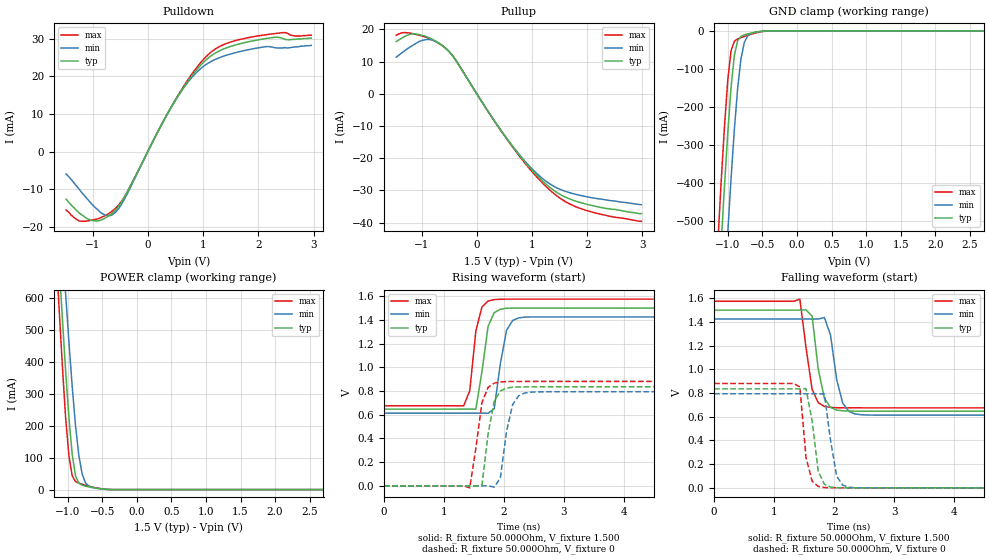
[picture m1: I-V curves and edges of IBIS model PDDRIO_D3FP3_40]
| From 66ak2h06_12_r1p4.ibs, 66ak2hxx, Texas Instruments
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|   Model PDDRIO_D3FP3_40
[Model] PDDRIO_D3FP3_40
Model_type   I/O
Polarity   Non-Inverting
Enable   Active-High
C_comp   3.236pF   3.174pF   3.318pF
C_comp_pullup   516.723fF   493.565fF   544.031fF
C_comp_pulldown 2.715pF   2.675pF   2.769pF
Vinh = 925.000mV
Vinl = 575.000mV
Vmeas = 750.000mV
Vref = 750.000mV
Rref = 50Ohms
Cref = 0pF
[Model Spec]
Vinh   925.000mV   888.000mV   963.000mV
Vinl   575.000mV   538.000mV   613.000mV
Vmeas   750.000mV   713.000mV   788.000mV
Vref   750.000mV   713.000mV   788.000mV
[Temperature Range]   25.000   125.000   -40.000
[Voltage Range]   1.500V   1.425V   1.575V
[GND Clamp Reference]   0.00V   0.00V   0.00V
|[C Comp Corner]
| variable   typ   min   max
|C_comp 3.236pF   3.318pF   3.174pF
|C_comp_pullup 516.723fF   544.031fF   493.565fF
|C_comp_pulldown 2.715pF   2.769pF   2.675pF
[Pulldown Reference]   0.00V   0.00V   0.00V
[POWER Clamp Reference]   1.500V   1.425V   1.575V
[Pullup Reference]   1.500V   1.425V   1.575V
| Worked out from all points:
|   slope of the pulldown table from 0 to 0.225 V, typ, clamps not added: 34.8 ohm
|   slope of the pullup table from 0 to 0.225 V, typ, clamps not added: 37.6 ohm
|   GND clamp passes 1 mA (typ) near -0.49 V on its own axis
|   POWER clamp passes 1 mA (typ) near -0.46 V on its own axis
|   rising waveform, R_fixture 50.000Ohm, V_fixture 1.500: 20-80 % time 145ps typ, 153ps min, 136ps max; typ from 0.647 V to 1.5 V
|   rising waveform, R_fixture 50.000Ohm, V_fixture 0: 20-80 % time 150ps typ, 158ps min, 147ps max; typ from 0 V to 0.836 V
|   falling waveform, R_fixture 50.000Ohm, V_fixture 1.500: 20-80 % time 151ps typ, 165ps min, 148ps max; typ from 1.5 V to 0.647 V
|   falling waveform, R_fixture 50.000Ohm, V_fixture 0: 20-80 % time 134ps typ, 143ps min, 118ps max; typ from 0.836 V to 0 V
[GND Clamp]
-1.48V    -1.918A    -2.181A    -1.764A
-1.145V   -723.4mA   -1.002A    -556.7mA
-1.098V   -563.3mA   -840.4mA   -399.2mA
-1.05V    -410.5mA   -683.3mA   -253.2mA
-1.002V   -269.5mA   -532mA     -130mA
-954.6mV  -149.1mA   -389.4mA   -52.57mA
-906.8mV  -64.77mA   -260.1mA   -27.53mA
-859.1mV  -26.06mA   -151.5mA   -21.41mA
-811.4mV  -14.61mA   -73.73mA   -17.98mA
-715.9mV  -8.245mA   -13.8mA    -12.04mA
-525mV    -1.646mA   -1.444mA   -2.745mA
2.959V    5.126nA    157.9nA    5.129nA
[Power Clamp]
-1.459V   2.052A     2.172A     2.008A
-1.173V   897.3mA    1.113A     766.5mA
-1.125V   714.9mA    943mA      572.9mA
-1.077V   539.1mA    776.9mA    390mA
-1.03V    373.7mA    616.2mA    227.4mA
-981.8mV  225.9mA    463.5mA    105.8mA
-934.1mV  109.7mA    322.9mA    43.29mA
-886.4mV  43.23mA    201.1mA    25.08mA
-838.6mV  20.27mA    107.7mA    20.03mA
-790.9mV  13.81mA    49.43mA    16.8mA
-647.7mV  6.613mA    6.926mA    8.545mA
2.98V     -9.151nA   -320.3nA   -14.09nA
[Pulldown]
-1.48V    -12.7mA    -6mA       -15.6mA
-1.241V   -16.4mA    -10.1mA    -18.5mA
-1.05V    -18.2mA    -13.4mA    -18.4mA
-811.4mV  -18.04mA   -16.66mA   -17.36mA
-668.2mV  -16.7mA    -17.04mA   -16.14mA
-381.8mV  -11.07mA   -11.53mA   -11.01mA
525mV     14.23mA    14.27mA    14.43mA
811.4mV   20.45mA    20mA       20.93mA
1.098V    24.97mA    23.6mA     25.9mA
1.384V    27.4mA     25.48mA    28.57mA
1.861V    29.38mA    27.26mA    30.48mA
2.959V    30.2mA     28.3mA     31mA
[Pullup]
-1.459V   16.2mA     11.34mA    18.17mA
-1.316V   17.7mA     13.24mA    19mA
-1.125V   18.6mA     15.39mA    18.51mA
-886.4mV  17.54mA    16.86mA    17.33mA
-695.5mV  15.85mA    15.81mA    15.72mA
-409.1mV  11.13mA    11.2mA     11.12mA
211.4mV   -5.637mA   -5.668mA   -5.687mA
640.9mV   -16.18mA   -16.11mA   -16.39mA
1.214V    -27.44mA   -26.64mA   -28.12mA
1.5V      -31.16mA   -29.62mA   -32.33mA
1.834V    -33.57mA   -31.39mA   -35.36mA
2.98V     -37.2mA    -34.46mA   -39.6mA
[Ramp]
R_load=50.000Ohm
dV/dt_r   506.520mV/133.500ps  481.679mV/142.000ps  534.210mV/125.000ps
dV/dt_f   506.520mV/123.500ps  481.679mV/133.500ps  534.210mV/115.500ps
[Rising waveform]
R_fixture=50.000Ohm
V_fixture=1.500
V_fixture_min=1.425
V_fixture_max=1.575
0s        647.2mV    613.5mV    675.3mV
1.327ns   647.3mV    613.5mV    675.3mV
1.429ns   647.3mV    613.5mV    800mV
1.531ns   647.3mV    613.5mV    1.306V
1.633ns   966mV      613.6mV    1.509V
1.735ns   1.346V     612.1mV    1.559V
1.837ns   1.461V     650.8mV    1.571V
2.042ns   1.498V     1.312V     1.575V
2.246ns   1.5V       1.417V     1.575V
10ns      1.5V       1.425V     1.575V
[Rising waveform]
R_fixture=50.000Ohm
V_fixture=0
0s        0V         2.011uV    0V
1.429ns   26.02uV    -4.175uV   -16.99mV
1.633ns   6.828mV    12.98uV    702.9mV
1.735ns   439.5mV    536.3uV    830.9mV
1.837ns   713.3mV    -10.93mV   866.4mV
1.939ns   799.8mV    66.69mV    876.4mV
2.042ns   825mV      460.5mV    879.5mV
2.144ns   832.1mV    686.1mV    880.5mV
2.348ns   835.1mV    783.6mV    880.9mV
10ns      835.6mV    794.1mV    881mV
[Falling waveform]
R_fixture=50.000Ohm
V_fixture=1.500
V_fixture_min=1.425
V_fixture_max=1.575
0s        1.5V       1.425V     1.575V
1.429ns   1.5V       1.425V     1.593V
1.633ns   1.45V      1.425V     832.5mV
1.735ns   1.003V     1.425V     718.7mV
1.837ns   756.6mV    1.438V     687.6mV
1.939ns   679.3mV    1.292V     679.2mV
2.042ns   656.7mV    913.6mV    676.5mV
2.144ns   650.4mV    713.8mV    675.7mV
2.348ns   647.6mV    623.6mV    675.4mV
10ns      647.2mV    613.5mV    675.3mV
[Falling waveform]
R_fixture=50.000Ohm
V_fixture=0
0s        835.6mV    794.1mV    881mV
1.429ns   835.6mV    794.1mV    851.5mV
1.531ns   837.3mV    794.1mV    258.9mV
1.633ns   566mV      794.2mV    56.51mV
1.735ns   139mV      794.1mV    12.14mV
1.837ns   31.44mV    792.5mV    2.563mV
1.939ns   7.085mV    403.7mV    527.9uV
2.042ns   1.539mV    97.55mV    88.32uV
2.246ns   66.01uV    5.292mV    1.05uV
10ns      0V         2.011uV    0V
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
